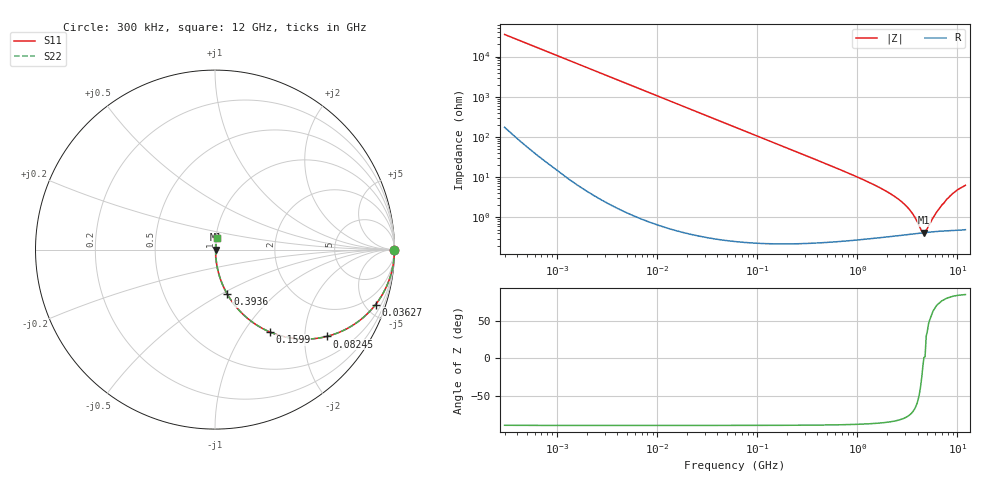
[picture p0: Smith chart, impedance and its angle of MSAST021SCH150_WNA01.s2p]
! MSAST021SCH150_WNA01  S-PARAMETER MODEL  ( General Type )
! Model Generated by TAIYO YUDEN Corporation (http://www.ty-top.com)
! Version 2.0
! TAIYO YUDEN Control No. 181101
! Copyright(c) 2016 TAIYO YUDEN CO.,LTD. All Rights Reserved.
! Product Description (link to TY-COMPAS)
! https://ds.yuden.co.jp/TYCOMPAS/or/detail?pn=MSAST021SCH150JWNA01&u=M
! Products Name : Multilayer Ceramic Capacitors
! Characteristics :
!  Capacitance : 15 pF , Rated Voltage : 25V , TCC : CH / C0H
!  Case Size : 0.25 x 0.125 / 0.0098 x 0.0049 [mm/inch] , Thickness : 0.125 / 0.0049 [mm/inch]
!  (Conditions: Temperature = 25 degC , DC Bias Current/Voltage = 0A / 0V)
! External Node Assignments :
!  1  o---| |---o  2
! GND o---------o GND
! Frequency Range : 0.3MHz  -  12000MHz  [ 401 STEP ]
# MHz S RI R 50
! Freq[MHz].  S11 Real  S11 Imag  S21 Real  S21 Imag  S12 Real  S12 Imag  S22 Real  S22 Imag
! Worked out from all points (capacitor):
!   401 points, 300 kHz to 12 GHz, reference 50 ohm
!   read as one part in series: C = 15 pF near 316.3 kHz
!   lowest |Z| = 417 mohm at 4.624 GHz (marker M1)
!   series resonance near 4.615 GHz, so ESL is about 79 pH
!   S11 on the Smith chart (normalised r, x): 300 kHz: open; 36.27 MHz: 1.01, -5.85; 82.45 MHz: 1.00, -2.57; 159.9 MHz: 1.00, -1.33; 393.6 MHz: 1.00, -0.54; 12 GHz: 1.01, +0.13
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0.3  1 -0.00283  2.19e-05 0.00283  2.19e-05 0.00283  1 -0.00283
1.769972  0.9997 -0.0167  0.000293 0.0167  0.000293 0.0167  0.9997 -0.0167
10.44266  0.9903 -0.0975  0.00965 0.0975  0.00965 0.0975  0.9903 -0.0975
36.27049  0.8951 -0.3059  0.1049 0.3059  0.1049 0.3059  0.8951 -0.3059
60  0.7573 -0.428  0.2427 0.428  0.2427 0.428  0.7573 -0.428
82.45425  0.6231 -0.4837  0.3769 0.4837  0.3769 0.4837  0.6231 -0.4837
159.8975  0.3058 -0.4591  0.6942 0.4591  0.6942 0.4591  0.3058 -0.4591
237.9135  0.1664 -0.3699  0.8336 0.3699  0.8336 0.3699  0.1664 -0.3699
353.9943  0.0833 -0.2725  0.9167 0.2725  0.9167 0.2725  0.0833 -0.2725
393.5654  0.0687 -0.2487  0.9313 0.2487  0.9313 0.2487  0.0687 -0.2487
1105.905  0.0108 -0.0891  0.9892 0.0891  0.9892 0.0891  0.0108 -0.0891
2088.533  0.00492 -0.0399  0.9951 0.0399  0.9951 0.0399  0.00492 -0.0399
2650.866  0.00425 -0.0265  0.9958 0.0265  0.9958 0.0265  0.00425 -0.0265
3190.978  0.00402 -0.017  0.996 0.017  0.996 0.017  0.00402 -0.017
3642.919  0.00399 -0.0107  0.996 0.0107  0.996 0.0107  0.00399 -0.0107
4385.161  0.0041 -0.00207  0.9959 0.00207  0.9959 0.00207  0.0041 -0.00207
4623.766  0.00416 7.02e-05  0.9958 -7.02e-05  0.9958 -7.02e-05  0.00416 7.02e-05
4875.354  0.00422 0.00242  0.9958 -0.00242  0.9958 -0.00242  0.00422 0.00242
6354.153  0.00468 0.014  0.9953 -0.014  0.9953 -0.014  0.00468 0.014
7854.144  0.00543 0.028  0.9946 -0.028  0.9946 -0.028  0.00543 0.028
9708.23  0.00684 0.0454  0.9932 -0.0454  0.9932 -0.0454  0.00684 0.0454
12000  0.00881 0.0619  0.9912 -0.0619  0.9912 -0.0619  0.00881 0.0619
